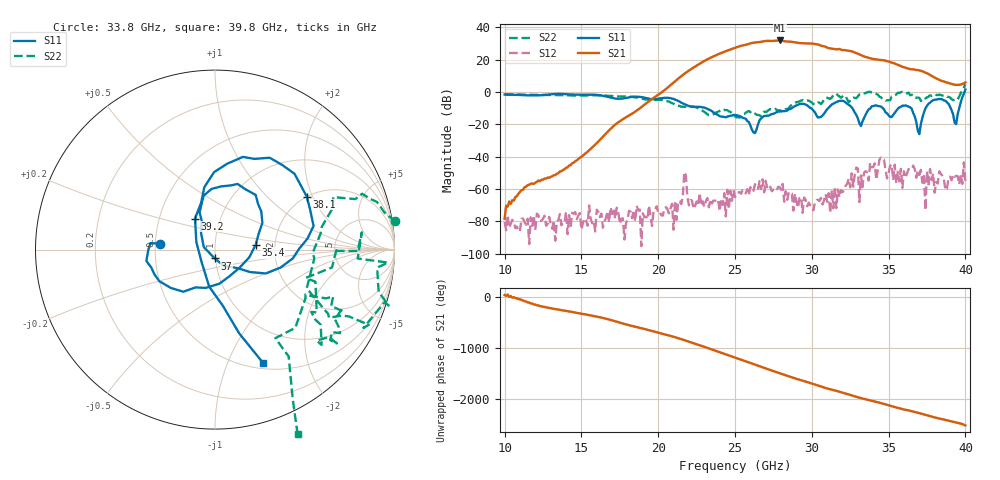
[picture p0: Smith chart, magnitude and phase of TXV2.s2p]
!Keysight Technologies,M9808A,MY58100618,A.14.70.03
!Date: Monday, February 27, 2023 13:37:26
!Correction: S11(C  2-Port  )
!S21(C  2-Port  )
!S12(C  2-Port  )
!S22(C  2-Port  )
!S2P File: Measurements: S11, S21, S12, S22:
# Hz S  RI  R 50
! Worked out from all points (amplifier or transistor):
!   301 points, 10 GHz to 40 GHz, reference 50 ohm
!   highest |S21| = 32.0 dB at 27.9 GHz (marker M1)
!   |S21| within 3 dB of that: 25.57 GHz to 30.55 GHz (4.975 GHz wide, 17.7 % of centre)
!   unconditionally stable (mu >= 1): start of sweep to 33.56 GHz; 34.11 GHz to 35.77 GHz; 35.95 GHz to 39.73 GHz
!   at 15 GHz: K = 112684.23, MAG = -31.0 dB, |S12| = -85.2 dB
!   at 25 GHz: K = 35.96, MAG = 27.6 dB, |S12| = -65.1 dB
!   at 40 GHz: K = 125.97, MSG = 30.6 dB, |S12| = -55.3 dB
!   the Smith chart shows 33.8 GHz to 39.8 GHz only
!   S11 on the Smith chart (normalised r, x): 33.8 GHz: 0.53, +0.04; 35.4 GHz: 1.58, +0.09; 37 GHz: 0.99, -0.10; 38.1 GHz: 2.00, +1.81; 39.2 GHz: 0.76, +0.27; 39.8 GHz: 0.57, -1.35
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1e10  0.6995 0.4627  9.45e-05 7.21e-05  -7.87e-05 -5.19e-05  0.0816 0.8402
1.5e10  0.6641 -0.4984  0.00847 0.00515  4.18e-05 -3.57e-05  0.7625 0.152
2e10  -0.1636 -0.5996  0.7697 0.2996  -2.51e-05 0.000181  0.2286 -0.5322
2.34e10  -0.255 -0.099  5.356 10.23  0.000401 0.000248  -0.0694 -0.1857
2.42e10  -0.1701 0.029  15.77 -6.211  0.000304 -9.97e-05  -0.1855 -0.2011
2.5e10  -0.1353 0.1421  -5.892 -22.47  0.000295 0.000472  -0.1379 -0.1127
2.59e10  -0.087 0.08  -29.1 10.37  0.000585 0.000274  -0.2466 0.0787
2.66e10  0.1296 -0.036  3.508 35.28  0.00138 0.00106  -0.1533 0.1154
2.73e10  0.1867 -0.07  37.61 6.475  0.00115 0.000141  -0.1079 0.2784
2.79e10  0.2003 -0.1494  23.9 -31.62  0.00104 0.000499  -0.0418 0.271
2.89e10  0.0666 -0.3617  -30.89 -16.49  0.000692 -0.000109  0.1907 0.4127
3e10  0.1212 -0.2795  -8.607 30.69  0.000165 0.000246  0.1726 0.442
3.09e10  -0.196 -0.1597  23.96 7.814  -0.000155 0.000671  0.6151 0.2515
3.21e10  -0.1657 -0.4892  3.397 -19.71  0.000154 0.000918  0.6449 0.4626
3.38e10  -0.306 0.0333  -8.111 7.726  0.00149 0.00627  1.005 0.157
3.5e10  0.025 -0.1897  6.764 5.738  -0.000704 -0.00311  0.511 -0.2157
3.54e10  0.2264 0.026  7.637 0.7959  -0.00497 0.00269  0.709 -0.3673
3.7e10  -0.000869 -0.0495  -1.815 -4.336  0.000976 0.00252  0.6517 -0.0995
3.81e10  0.5112 0.2954  -2.412 1.101  -0.00129 0.00102  0.642 -0.5049
3.92e10  -0.1113 0.1728  0.3239 1.697  -0.00258 -0.00103  0.5031 -0.2504
3.98e10  0.2683 -0.6317  1.497 0.9654  -0.00142 0.000206  0.4603 -1.029
4e10  0.6193 -1.026  1.982 0.2108  -0.0012 0.00124  0.7451 -1.559
